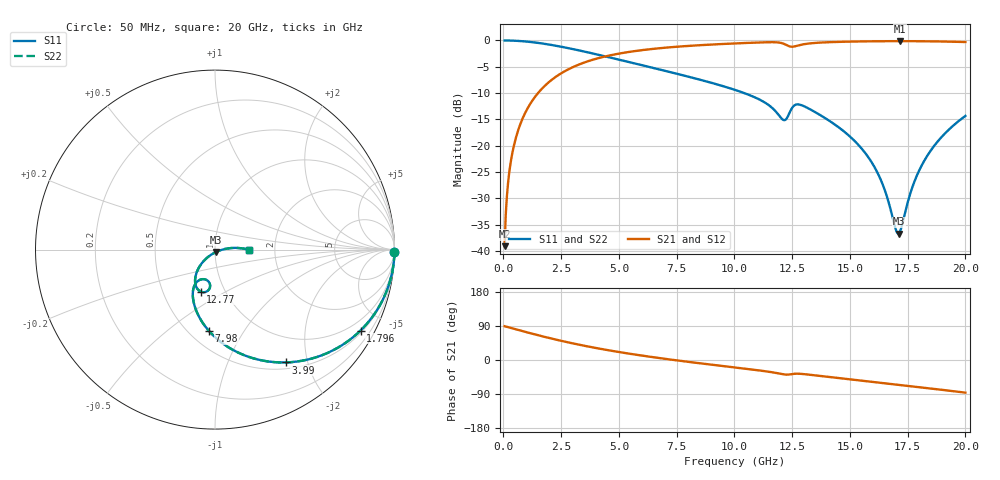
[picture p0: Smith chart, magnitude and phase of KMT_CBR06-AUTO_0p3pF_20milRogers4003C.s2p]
! Data measured by Modelithics Inc. support@modelithics.com 813-866-6335
! KEMET CBR06-AUTO 0.3pF, Pad Width= 0.851mm, Pad Length= 0.64mm, Pad Gap= 0.62mm, 20mil Rogers 4003C substrate Data, January 2022
# hz S ma R 50
! 2 Port Network Data from SP1.SP block
! freq  magS11  angS11  magS21  angS21  magS12  angS12  magS22  angS22
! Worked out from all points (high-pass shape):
!   401 points, 50 MHz to 20 GHz, reference 50 ohm
!   highest |S21| = -0.13 dB at 17.16 GHz (marker M1); lowest = -39.1 dB at 50 MHz (marker M2)
!   |S21| within 3 dB of the highest: 4.315 GHz to end of sweep
!   lowest |S11| = -36.7 dB at 17.11 GHz (marker M3), VSWR 1.03, Z = 50.7 - j1.31 ohm
!   |S11| at or under -10 dB: 10.43 GHz to end of sweep
!   |S22| runs from -36.7 to 0.0 dB; largest |S21 - S12| = 0
!   S11 on the Smith chart (normalised r, x): 50 MHz: open; 1.796 GHz: 0.58, -3.77; 3.99 GHz: 0.59, -1.65; 7.98 GHz: 0.62, -0.71; 12.77 GHz: 0.77, -0.38; 20 GHz: 1.48, -0.01
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5e7  0.9999 -0.8  0.01113 89.2  0.01113 89.2  0.9999 -0.8
2.495e8  0.9984 -4.2  0.05547 85.8  0.05547 85.8  0.9984 -4.2
5.4875e8  0.9925 -9.2  0.1213 80.8  0.1213 80.8  0.9925 -9.2
1.0475e9  0.9736 -17.4  0.2273 72.6  0.2273 72.6  0.9736 -17.4
1.795625e9  0.9276 -29.1  0.3718 60.8  0.3718 60.8  0.9276 -29.1
3.391625e9  0.7939 -50.9  0.6052 38.9  0.6052 38.9  0.7939 -50.9
3.990125e9  0.7415 -58.0  0.6679 31.8  0.6679 31.8  0.7415 -58.0
6.73325e9  0.532 -84.4  0.8429 5.2  0.8429 5.2  0.532 -84.4
7.980125e9  0.4545 -94.2  0.8868 -4.7  0.8868 -4.7  0.4545 -94.2
1.0025e10  0.3394 -109.2  0.937 -19.7  0.937 -19.7  0.3394 -109.2
1.132175e10  0.257 -118.4  0.9607 -29.6  0.9607 -29.6  0.257 -118.4
1.211975e10  0.1757 -110.3  0.9329 -37.8  0.9329 -37.8  0.1757 -110.3
1.276812e10  0.247 -108.7  0.8974 -36.2  0.8974 -36.2  0.247 -108.7
1.336662e10  0.2165 -120.7  0.9426 -39.6  0.9426 -39.6  0.2165 -120.7
1.556112e10  0.09109 -134.7  0.9796 -54.7  0.9796 -54.7  0.09109 -134.7
1.62095e10  0.05463 -133.1  0.983 -59.1  0.983 -59.1  0.05463 -133.1
1.670825e10  0.02747 -120.1  0.9844 -62.6  0.9844 -62.6  0.02747 -120.1
1.710725e10  0.01463 -62.1  0.9848 -65.3  0.9848 -65.3  0.01463 -62.1
1.715712e10  0.0151 -50.8  0.9848 -65.7  0.9848 -65.7  0.0151 -50.8
1.770575e10  0.04053 -0.5  0.9842 -69.5  0.9842 -69.5  0.04053 -0.5
1.82045e10  0.07114 5.2  0.9825 -73.1  0.9825 -73.1  0.07114 5.2
2e10  0.1921 -0.7  0.9659 -86.2  0.9659 -86.2  0.1921 -0.7
